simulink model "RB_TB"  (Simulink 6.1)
settings: Solver=ode3  SolverMode=SingleTasking  StartTime=0  StopTime=0.1  FixedStep=0.01  RelTol=1e-3
libraries: simulink x2
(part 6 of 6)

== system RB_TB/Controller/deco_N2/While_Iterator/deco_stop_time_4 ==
  note: Model: RB_TB/Controller/deco_N2/While_Iterator/deco_stop_time_X
  bus1 : Inport  Port=1  LatchInput=off
  bus2 : Inport  Port=2  LatchInput=off
  >10e-300 : Saturate  UpperLimit=inf  LowerLimit=10e-320
  >10e-320 : Switch  Threshold=10e-320
  BS1 : BusSelector  DialogController=Simulink.DDGSource_Bus  OutputSignals=N2_k,Pt_stop,N2_b,M0
  BS2 : BusSelector  DialogController=Simulink.DDGSource_Bus  OutputSignals=Pstop_next,Palv_next,stop_time
  Constant : Constant
  Mem : Memory  InheritSampleTime=on
  Mux1 : Mux  Inputs=2
  Mux2 : Mux
  Mux3 : Mux  Inputs=2
  Mux4 : Mux  Inputs=3
  Mux5 : Mux  Inputs=3
  fcn(14)1 : Fcn  Expr=log(u(1))
  fcn(14)4 : Fcn  Expr=u(1)-u(2)
  fcn(14)5 : Fcn  Expr=-u(2)/u(1)
  fcn(14)6 : Fcn  Expr=(u(2)-u(3))/u(1)
  fcn1 : Fcn  Expr=u(2)+u(3)/u(1)
  fcn2 : Fcn  Expr=u(3)+(u(2)-u(3))*exp(-u(1)*u(4))
  Pt_new : Outport
  deco_stop_time : Outport  Port=2
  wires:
  >10e-300/1 -> Mux5/1
  Mux5/1 -> fcn(14)6/1
  fcn(14)4/1 -> >10e-300/1
  Mux3/1 -> fcn(14)4/1
  fcn(14)6/1 -> >10e-320/1, >10e-320/2
  fcn1/1 -> Mux5/2  "M_next"
  bus2/1 -> BS2/1
  Mem/1 -> Pt_new/1
  BS2/3 -> Mux2/4  "<stop_time>"
  fcn2/1 -> Mem/1
  Mux2/1 -> fcn2/1
  BS1/2 -> Mux3/1, Mux2/2  "<Pt_stop>"
  BS2/1 -> Mux4/3  "<Pstop_next>"
  bus1/1 -> BS1/1
  BS1/3 -> Mux4/1  "<N2_b>"
  BS1/4 -> Mux4/2  "<M0>"
  Mux1/1 -> fcn(14)5/1
  BS1/1 -> Mux2/1, Mux1/1  "<N2_k>"
  BS2/2 -> Mux5/3, Mux2/3, Mux3/2  "<Palv_next>"
  fcn(14)5/1 -> deco_stop_time/1  "deco_stop_time"
  Mux4/1 -> fcn1/1
  >10e-320/1 -> fcn(14)1/1
  fcn(14)1/1 -> Mux1/2
  Constant/1 -> >10e-320/3

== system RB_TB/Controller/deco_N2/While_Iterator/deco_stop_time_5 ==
  note: Model: RB_TB/Controller/deco_N2/While_Iterator/deco_stop_time_X
  bus1 : Inport  Port=1  LatchInput=off
  bus2 : Inport  Port=2  LatchInput=off
  >10e-300 : Saturate  UpperLimit=inf  LowerLimit=10e-320
  >10e-320 : Switch  Threshold=10e-320
  BS1 : BusSelector  DialogController=Simulink.DDGSource_Bus  OutputSignals=N2_k,Pt_stop,N2_b,M0
  BS2 : BusSelector  DialogController=Simulink.DDGSource_Bus  OutputSignals=Pstop_next,Palv_next,stop_time
  Constant : Constant
  Mem : Memory  InheritSampleTime=on
  Mux1 : Mux  Inputs=2
  Mux2 : Mux
  Mux3 : Mux  Inputs=2
  Mux4 : Mux  Inputs=3
  Mux5 : Mux  Inputs=3
  fcn(14)1 : Fcn  Expr=log(u(1))
  fcn(14)4 : Fcn  Expr=u(1)-u(2)
  fcn(14)5 : Fcn  Expr=-u(2)/u(1)
  fcn(14)6 : Fcn  Expr=(u(2)-u(3))/u(1)
  fcn1 : Fcn  Expr=u(2)+u(3)/u(1)
  fcn2 : Fcn  Expr=u(3)+(u(2)-u(3))*exp(-u(1)*u(4))
  Pt_new : Outport
  deco_stop_time : Outport  Port=2
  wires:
  Constant/1 -> >10e-320/3
  fcn(14)1/1 -> Mux1/2
  >10e-320/1 -> fcn(14)1/1
  Mux4/1 -> fcn1/1
  fcn(14)5/1 -> deco_stop_time/1  "deco_stop_time"
  BS2/2 -> Mux3/2, Mux2/3, Mux5/3  "<Palv_next>"
  BS1/1 -> Mux1/1, Mux2/1  "<N2_k>"
  Mux1/1 -> fcn(14)5/1
  BS1/4 -> Mux4/2  "<M0>"
  BS1/3 -> Mux4/1  "<N2_b>"
  bus1/1 -> BS1/1
  BS2/1 -> Mux4/3  "<Pstop_next>"
  BS1/2 -> Mux2/2, Mux3/1  "<Pt_stop>"
  Mux2/1 -> fcn2/1
  fcn2/1 -> Mem/1
  BS2/3 -> Mux2/4  "<stop_time>"
  Mem/1 -> Pt_new/1
  bus2/1 -> BS2/1
  fcn1/1 -> Mux5/2  "M_next"
  fcn(14)6/1 -> >10e-320/2, >10e-320/1
  Mux3/1 -> fcn(14)4/1
  fcn(14)4/1 -> >10e-300/1
  Mux5/1 -> fcn(14)6/1
  >10e-300/1 -> Mux5/1

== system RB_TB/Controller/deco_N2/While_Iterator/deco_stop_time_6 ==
  note: Model: RB_TB/Controller/deco_N2/While_Iterator/deco_stop_time_X
  bus1 : Inport  Port=1  LatchInput=off
  bus2 : Inport  Port=2  LatchInput=off
  >10e-300 : Saturate  UpperLimit=inf  LowerLimit=10e-320
  >10e-320 : Switch  Threshold=10e-320
  BS1 : BusSelector  DialogController=Simulink.DDGSource_Bus  OutputSignals=N2_k,Pt_stop,N2_b,M0
  BS2 : BusSelector  DialogController=Simulink.DDGSource_Bus  OutputSignals=Pstop_next,Palv_next,stop_time
  Constant : Constant
  Mem : Memory  InheritSampleTime=on
  Mux1 : Mux  Inputs=2
  Mux2 : Mux
  Mux3 : Mux  Inputs=2
  Mux4 : Mux  Inputs=3
  Mux5 : Mux  Inputs=3
  fcn(14)1 : Fcn  Expr=log(u(1))
  fcn(14)4 : Fcn  Expr=u(1)-u(2)
  fcn(14)5 : Fcn  Expr=-u(2)/u(1)
  fcn(14)6 : Fcn  Expr=(u(2)-u(3))/u(1)
  fcn1 : Fcn  Expr=u(2)+u(3)/u(1)
  fcn2 : Fcn  Expr=u(3)+(u(2)-u(3))*exp(-u(1)*u(4))
  Pt_new : Outport
  deco_stop_time : Outport  Port=2
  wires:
  >10e-300/1 -> Mux5/1
  Mux5/1 -> fcn(14)6/1
  fcn(14)4/1 -> >10e-300/1
  Mux3/1 -> fcn(14)4/1
  fcn(14)6/1 -> >10e-320/1, >10e-320/2
  fcn1/1 -> Mux5/2  "M_next"
  bus2/1 -> BS2/1
  Mem/1 -> Pt_new/1
  BS2/3 -> Mux2/4  "<stop_time>"
  fcn2/1 -> Mem/1
  Mux2/1 -> fcn2/1
  BS1/2 -> Mux3/1, Mux2/2  "<Pt_stop>"
  BS2/1 -> Mux4/3  "<Pstop_next>"
  bus1/1 -> BS1/1
  BS1/3 -> Mux4/1  "<N2_b>"
  BS1/4 -> Mux4/2  "<M0>"
  Mux1/1 -> fcn(14)5/1
  BS1/1 -> Mux2/1, Mux1/1  "<N2_k>"
  BS2/2 -> Mux5/3, Mux2/3, Mux3/2  "<Palv_next>"
  fcn(14)5/1 -> deco_stop_time/1  "deco_stop_time"
  Mux4/1 -> fcn1/1
  >10e-320/1 -> fcn(14)1/1
  fcn(14)1/1 -> Mux1/2
  Constant/1 -> >10e-320/3

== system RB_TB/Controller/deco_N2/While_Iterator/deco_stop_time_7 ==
  note: Model: RB_TB/Controller/deco_N2/While_Iterator/deco_stop_time_X
  bus1 : Inport  Port=1  LatchInput=off
  bus2 : Inport  Port=2  LatchInput=off
  >10e-300 : Saturate  UpperLimit=inf  LowerLimit=10e-320
  >10e-320 : Switch  Threshold=10e-320
  BS1 : BusSelector  DialogController=Simulink.DDGSource_Bus  OutputSignals=N2_k,Pt_stop,N2_b,M0
  BS2 : BusSelector  DialogController=Simulink.DDGSource_Bus  OutputSignals=Pstop_next,Palv_next,stop_time
  Constant : Constant
  Mem : Memory  InheritSampleTime=on
  Mux1 : Mux  Inputs=2
  Mux2 : Mux
  Mux3 : Mux  Inputs=2
  Mux4 : Mux  Inputs=3
  Mux5 : Mux  Inputs=3
  fcn(14)1 : Fcn  Expr=log(u(1))
  fcn(14)4 : Fcn  Expr=u(1)-u(2)
  fcn(14)5 : Fcn  Expr=-u(2)/u(1)
  fcn(14)6 : Fcn  Expr=(u(2)-u(3))/u(1)
  fcn1 : Fcn  Expr=u(2)+u(3)/u(1)
  fcn2 : Fcn  Expr=u(3)+(u(2)-u(3))*exp(-u(1)*u(4))
  Pt_new : Outport
  deco_stop_time : Outport  Port=2
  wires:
  Constant/1 -> >10e-320/3
  fcn(14)1/1 -> Mux1/2
  >10e-320/1 -> fcn(14)1/1
  Mux4/1 -> fcn1/1
  fcn(14)5/1 -> deco_stop_time/1  "deco_stop_time"
  BS2/2 -> Mux3/2, Mux2/3, Mux5/3  "<Palv_next>"
  BS1/1 -> Mux1/1, Mux2/1  "<N2_k>"
  Mux1/1 -> fcn(14)5/1
  BS1/4 -> Mux4/2  "<M0>"
  BS1/3 -> Mux4/1  "<N2_b>"
  bus1/1 -> BS1/1
  BS2/1 -> Mux4/3  "<Pstop_next>"
  BS1/2 -> Mux2/2, Mux3/1  "<Pt_stop>"
  Mux2/1 -> fcn2/1
  fcn2/1 -> Mem/1
  BS2/3 -> Mux2/4  "<stop_time>"
  Mem/1 -> Pt_new/1
  bus2/1 -> BS2/1
  fcn1/1 -> Mux5/2  "M_next"
  fcn(14)6/1 -> >10e-320/2, >10e-320/1
  Mux3/1 -> fcn(14)4/1
  fcn(14)4/1 -> >10e-300/1
  Mux5/1 -> fcn(14)6/1
  >10e-300/1 -> Mux5/1

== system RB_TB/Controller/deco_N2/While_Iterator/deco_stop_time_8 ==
  note: Model: RB_TB/Controller/deco_N2/While_Iterator/deco_stop_time_X
  bus1 : Inport  Port=1  LatchInput=off
  bus2 : Inport  Port=2  LatchInput=off
  >10e-300 : Saturate  UpperLimit=inf  LowerLimit=10e-320
  >10e-320 : Switch  Threshold=10e-320
  BS1 : BusSelector  DialogController=Simulink.DDGSource_Bus  OutputSignals=N2_k,Pt_stop,N2_b,M0
  BS2 : BusSelector  DialogController=Simulink.DDGSource_Bus  OutputSignals=Pstop_next,Palv_next,stop_time
  Constant : Constant
  Mem : Memory  InheritSampleTime=on
  Mux1 : Mux  Inputs=2
  Mux2 : Mux
  Mux3 : Mux  Inputs=2
  Mux4 : Mux  Inputs=3
  Mux5 : Mux  Inputs=3
  fcn(14)1 : Fcn  Expr=log(u(1))
  fcn(14)4 : Fcn  Expr=u(1)-u(2)
  fcn(14)5 : Fcn  Expr=-u(2)/u(1)
  fcn(14)6 : Fcn  Expr=(u(2)-u(3))/u(1)
  fcn1 : Fcn  Expr=u(2)+u(3)/u(1)
  fcn2 : Fcn  Expr=u(3)+(u(2)-u(3))*exp(-u(1)*u(4))
  Pt_new : Outport
  deco_stop_time : Outport  Port=2
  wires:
  >10e-300/1 -> Mux5/1
  Mux5/1 -> fcn(14)6/1
  fcn(14)4/1 -> >10e-300/1
  Mux3/1 -> fcn(14)4/1
  fcn(14)6/1 -> >10e-320/1, >10e-320/2
  fcn1/1 -> Mux5/2  "M_next"
  bus2/1 -> BS2/1
  Mem/1 -> Pt_new/1
  BS2/3 -> Mux2/4  "<stop_time>"
  fcn2/1 -> Mem/1
  Mux2/1 -> fcn2/1
  BS1/2 -> Mux3/1, Mux2/2  "<Pt_stop>"
  BS2/1 -> Mux4/3  "<Pstop_next>"
  bus1/1 -> BS1/1
  BS1/3 -> Mux4/1  "<N2_b>"
  BS1/4 -> Mux4/2  "<M0>"
  Mux1/1 -> fcn(14)5/1
  BS1/1 -> Mux2/1, Mux1/1  "<N2_k>"
  BS2/2 -> Mux5/3, Mux2/3, Mux3/2  "<Palv_next>"
  fcn(14)5/1 -> deco_stop_time/1  "deco_stop_time"
  Mux4/1 -> fcn1/1
  >10e-320/1 -> fcn(14)1/1
  fcn(14)1/1 -> Mux1/2
  Constant/1 -> >10e-320/3

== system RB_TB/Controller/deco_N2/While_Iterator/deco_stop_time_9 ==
  note: Model: RB_TB/Controller/deco_N2/While_Iterator/deco_stop_time_X
  bus1 : Inport  Port=1  LatchInput=off
  bus2 : Inport  Port=2  LatchInput=off
  >10e-300 : Saturate  UpperLimit=inf  LowerLimit=10e-320
  >10e-320 : Switch  Threshold=10e-320
  BS1 : BusSelector  DialogController=Simulink.DDGSource_Bus  OutputSignals=N2_k,Pt_stop,N2_b,M0
  BS2 : BusSelector  DialogController=Simulink.DDGSource_Bus  OutputSignals=Pstop_next,Palv_next,stop_time
  Constant : Constant
  Mem : Memory  InheritSampleTime=on
  Mux1 : Mux  Inputs=2
  Mux2 : Mux
  Mux3 : Mux  Inputs=2
  Mux4 : Mux  Inputs=3
  Mux5 : Mux  Inputs=3
  fcn(14)1 : Fcn  Expr=log(u(1))
  fcn(14)4 : Fcn  Expr=u(1)-u(2)
  fcn(14)5 : Fcn  Expr=-u(2)/u(1)
  fcn(14)6 : Fcn  Expr=(u(2)-u(3))/u(1)
  fcn1 : Fcn  Expr=u(2)+u(3)/u(1)
  fcn2 : Fcn  Expr=u(3)+(u(2)-u(3))*exp(-u(1)*u(4))
  Pt_new : Outport
  deco_stop_time : Outport  Port=2
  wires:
  Constant/1 -> >10e-320/3
  fcn(14)1/1 -> Mux1/2
  >10e-320/1 -> fcn(14)1/1
  Mux4/1 -> fcn1/1
  fcn(14)5/1 -> deco_stop_time/1  "deco_stop_time"
  BS2/2 -> Mux3/2, Mux2/3, Mux5/3  "<Palv_next>"
  BS1/1 -> Mux1/1, Mux2/1  "<N2_k>"
  Mux1/1 -> fcn(14)5/1
  BS1/4 -> Mux4/2  "<M0>"
  BS1/3 -> Mux4/1  "<N2_b>"
  bus1/1 -> BS1/1
  BS2/1 -> Mux4/3  "<Pstop_next>"
  BS1/2 -> Mux2/2, Mux3/1  "<Pt_stop>"
  Mux2/1 -> fcn2/1
  fcn2/1 -> Mem/1
  BS2/3 -> Mux2/4  "<stop_time>"
  Mem/1 -> Pt_new/1
  bus2/1 -> BS2/1
  fcn1/1 -> Mux5/2  "M_next"
  fcn(14)6/1 -> >10e-320/2, >10e-320/1
  Mux3/1 -> fcn(14)4/1
  fcn(14)4/1 -> >10e-300/1
  Mux5/1 -> fcn(14)6/1
  >10e-300/1 -> Mux5/1
